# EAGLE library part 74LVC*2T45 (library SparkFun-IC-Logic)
Nexperia Dual Supply Translating Transceiver The 74LVC2T45 and 74LVCH2T45 are dual bit, dual supply translating transceivers with 3-state outputs that enable bidirectional level translation. They feature two 2-bits input-output ports (nA and nB), a direction control input (DIR) and dual supply pins (VCC(A) and VCC(B)). Both VCC(A) and VCC(B) can be supplied at any voltage between 1.2 V and 5.5 V making the device suitable for translating between any of the low voltage nodes (1.2 V, 1.5 V, 1.8 V, 2.5 V, 3.3 V and 5.0 V). Pins nA and DIR are referenced to VCC(A) and pins nB are referenced to VCC(B). A HIGH on DIR allows transmission from nA to nB and a LOW on DIR allows transmission from nB to nA. Datasheet
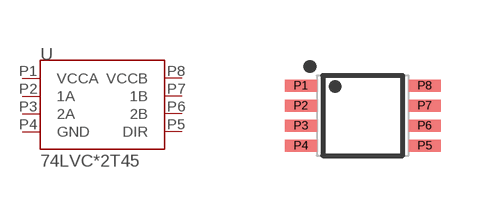
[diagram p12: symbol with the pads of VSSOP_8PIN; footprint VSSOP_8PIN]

Designator prefix U

## 74LVC2T45  [VSSOP_8PIN]
P1  VCCA
P2  1A
P3  2A
P4  GND
P5  DIR
P6  2B
P7  1B
P8  VCCB

## Footprint VSSOP_8PIN (pad centres in mm)
VSSOP 8-Pin Physical Characteristics Lead to Lead SIze: 3.2 x 2.1 mm Body Size: 2.1 x 2.4 x .9 mm Lead: .25 x .8 mm Pitch: .5 mm
smd 0.8 x 0.3: P1 -1.55,0.75; P2 -1.55,0.25; P3 -1.55,-0.25; P4 -1.55,-0.75; P5 1.55,-0.75; P6 1.55,-0.25; P7 1.55,0.25; P8 1.55,0.75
